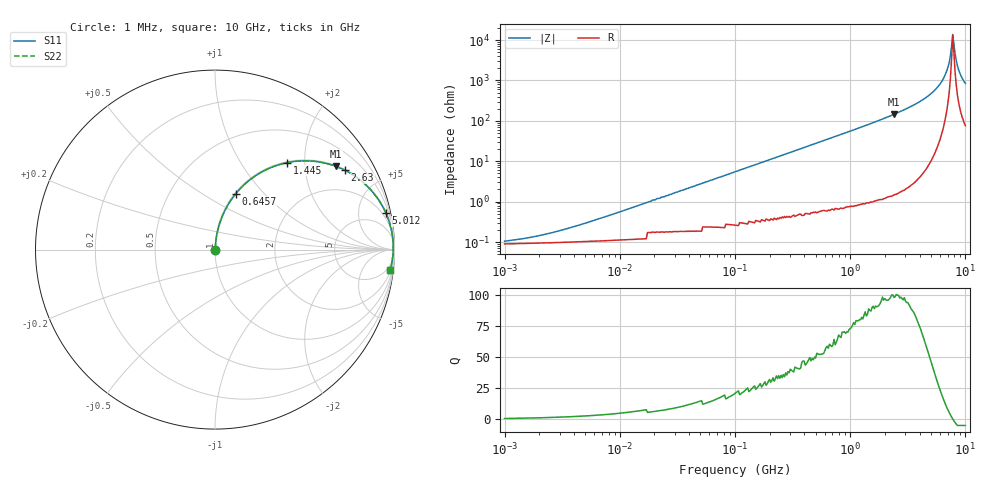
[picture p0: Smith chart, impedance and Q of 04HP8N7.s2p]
# MHz S MA R 50
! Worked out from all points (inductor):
!   401 points, 1 MHz to 10 GHz, reference 50 ohm
!   read as one part in series: L = 8.7 nH near 5.754 MHz
!   highest Q = 100 at 2.399 GHz (marker M1), where L = 9.62 nH
!   self-resonance near 7.762 GHz
!   S11 on the Smith chart (normalised r, x): 1 MHz: 1.00, +0.00; 645.7 MHz: 1.01, +0.71; 1.445 GHz: 1.02, +1.64; 2.63 GHz: 1.03, +3.25; 5.012 GHz: 1.18, +9.35; 10 GHz: 2, -17
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1  0.0009624 34.5  0.999 -0.0  0.999 -0.0  0.0009624 34.5
2.042  0.001423 51.5  0.999 -0.1  0.999 -0.1  0.001423 51.5
4.677  0.002758 67.7  0.999 -0.1  0.999 -0.1  0.002758 67.7
21.878  0.012 81.8  0.998 -0.7  0.998 -0.7  0.012 81.8
102.329  0.056 84.0  0.996 -3.2  0.996 -3.2  0.056 84.0
467.735  0.247 74.5  0.964 -14.3  0.964 -14.3  0.247 74.5
645.654  0.333 69.6  0.937 -19.5  0.937 -19.5  0.333 69.6
1445.44  0.63 50.3  0.77 -39.0  0.77 -39.0  0.63 50.3
2187.762  0.788 37.4  0.607 -52.0  0.607 -52.0  0.788 37.4
2398.833  0.819 34.4  0.565 -55.0  0.565 -55.0  0.819 34.4
2630.268  0.848 31.5  0.522 -57.9  0.522 -57.9  0.848 31.5
3801.894  0.935 20.0  0.343 -69.2  0.343 -69.2  0.935 20.0
5011.872  0.974 12.0  0.208 -76.8  0.208 -76.8  0.974 12.0
5888.437  0.986 7.5  0.131 -80.3  0.131 -80.3  0.986 7.5
6606.934  0.991 4.4  0.077 -81.4  0.077 -81.4  0.991 4.4
7079.458  0.993 2.6  0.045 -79.6  0.045 -79.6  0.993 2.6
7413.102  0.993 1.3  0.024 -72.8  0.024 -72.8  0.993 1.3
7762.471  0.993 0.1  0.00722 -13.5  0.00722 -13.5  0.993 0.1
8128.305  0.992 -1.1  0.021 68.0  0.021 68.0  0.992 -1.1
8511.38  0.991 -2.4  0.042 76.5  0.042 76.5  0.991 -2.4
8912.509  0.989 -3.6  0.063 78.5  0.063 78.5  0.989 -3.6
10000  0.983 -6.7  0.117 78.1  0.117 78.1  0.983 -6.7
